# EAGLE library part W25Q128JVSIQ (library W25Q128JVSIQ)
128M-bit Serial Flash Memory with uniform 4KB sectors and Dual/Quad SPI Source: Datasheet
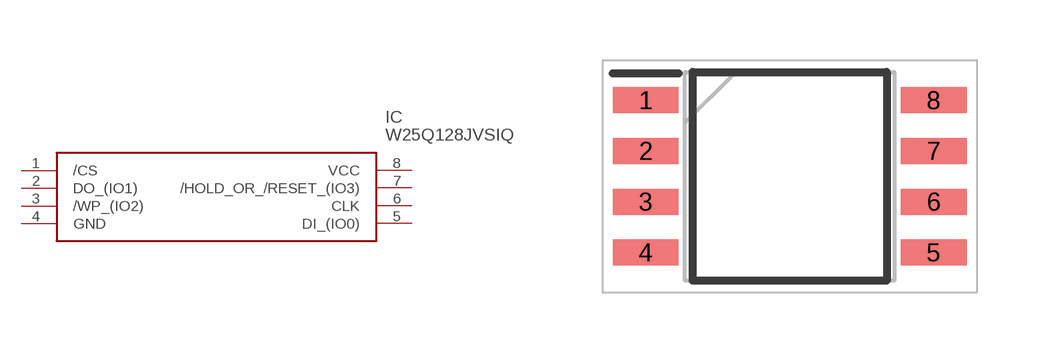
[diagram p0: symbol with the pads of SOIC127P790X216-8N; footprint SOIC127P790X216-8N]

Designator prefix IC

## W25Q128JVSIQ (Description: 128M-bit Serial Flash Memory with uniform 4KB sectors and Dual/Quad SPI; Height: 2.16mm; Manufacturer_Name: Winbond; Manufacturer_Part_Number: W25Q128JVSIQ; Mouser_Part_Number: 454-W25Q128JVSIQ; Mouser_Price-Stock: https://www.mouser.co.uk/ProductDetail/Winbond/W25Q128JVSIQ?qs=qSfuJ%252Bfl%2Fd6tLXvPR4fl9w%3D%3D)  [SOIC127P790X216-8N]
1  /CS
2  DO_(IO1)
3  /WP_(IO2)
4  GND
5  DI_(IO0)
6  CLK
7  /HOLD_OR_/RESET_(IO3)
8  VCC

## Footprint SOIC127P790X216-8N (pad centres in mm)
W25Q128JVSIQ
smd 1.65 x 0.65: 1 -3.6,1.905; 2 -3.6,0.635; 3 -3.6,-0.635; 4 -3.6,-1.905; 5 3.6,-1.905; 6 3.6,-0.635; 7 3.6,0.635; 8 3.6,1.905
